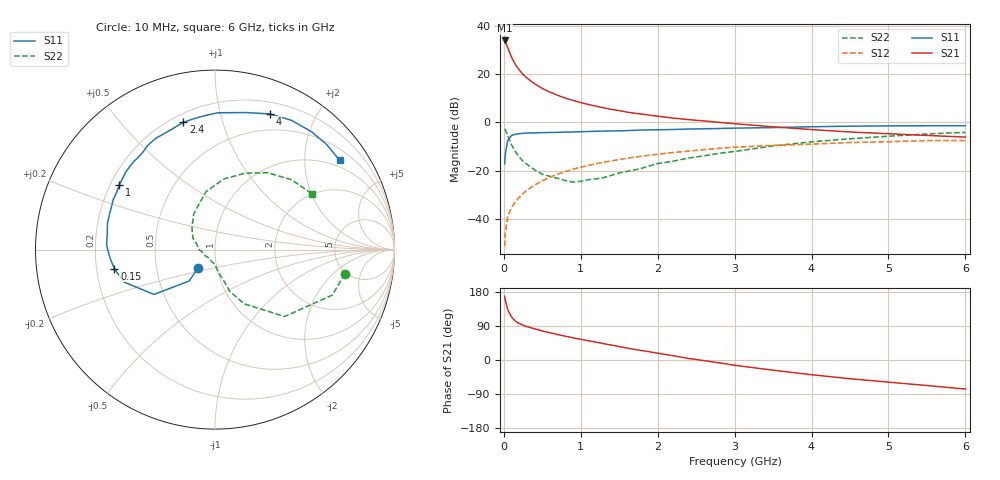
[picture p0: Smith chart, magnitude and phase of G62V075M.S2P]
! SIEMENS Small Signal Semiconductors
! BFG193
! Si NPN RF Bipolar Junction Transistor in SOT223
! VCE = 2 V  IC = 75 mA
! Common Emitter S-Parameters:  August  1996
# GHz  S  MA  R  50
!  f  S11  S21  S12  S22
! GHz  MAG  ANG  MAG  ANG  MAG  ANG  MAG  ANG
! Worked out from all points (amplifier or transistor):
!   36 points, 10 MHz to 6 GHz, reference 50 ohm
!   highest |S21| = 34.1 dB at 10 MHz (marker M1)
!   |S21| within 3 dB of that: start of sweep to 50.66 MHz
!   unconditionally stable (mu >= 1): start of sweep to 18.9 MHz; 178.8 MHz to 2.977 GHz; 3.075 GHz to 3.645 GHz
!   at 250 MHz: K = 1.06, MAG = 23.3 dB, |S12| = -29.5 dB
!   at 1.4 GHz: K = 1.11, MAG = 8.7 dB, |S12| = -16.0 dB
!   at 6 GHz: K = 1.00, MSG = 0.7 dB, |S12| = -7.5 dB
!   S11 on the Smith chart (normalised r, x): 10 MHz: 0.81, -0.17; 150 MHz: 0.28, -0.09; 1 GHz: 0.24, +0.29; 2.4 GHz: 0.25, +0.75; 4 GHz: 0.32, +1.43; 6 GHz: 0.79, +2.92
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0.01  0.1376 -132.7  50.46 168.0  0.0027 73.3  0.7358 -10.5
0.02  0.2262 -129.4  47.25 157.3  0.0052 72.5  0.701 -21.2
0.05  0.422 -143.7  35.94 132.8  0.0112 63.2  0.5379 -43.9
0.1  0.5383 -160.4  22.73 113.3  0.0171 64.5  0.3431 -61.7
0.15  0.5708 -169.3  15.97 102.5  0.0225 65.2  0.2467 -70.5
0.2  0.5852 -174.9  12.34 96.5  0.0278 66.9  0.1937 -73.1
0.25  0.5959 -179.2  9.963 91.8  0.0334 67.6  0.1557 -77.1
0.3  0.6044 177.4  8.381 88.2  0.0391 68.9  0.1357 -80.1
0.4  0.6069 171.3  6.34 82.3  0.0502 69.4  0.1035 -85.2
0.5  0.6166 166.4  5.086 76.6  0.0615 68.2  0.0843 -89.8
0.6  0.6197 161.9  4.269 71.8  0.0732 67.0  0.0758 -95.8
0.8  0.6317 154.0  3.21 62.7  0.0956 63.4  0.0622 -116.4
1  0.6438 145.8  2.589 54.5  0.1176 59.5  0.06 -136.4
1.1  0.6496 142.4  2.362 50.7  0.1282 57.7  0.0649 -147.5
1.6  0.6775 125.9  1.644 31.6  0.18 46.1  0.0966 171.9
2.2  0.7144 109.0  1.233 11.3  0.2373 31.7  0.1567 143.8
2.4  0.7307 103.9  1.146 4.3  0.2546 27.3  0.1828 134.5
3.5  0.7828 77.3  0.813 -26.9  0.3337 -0.9  0.3254 99.1
4  0.8154 68.0  0.713 -38.8  0.3554 -10.8  0.3969 82.9
4.5  0.8372 59.3  0.634 -49.4  0.3832 -21.1  0.4585 68.3
5.5  0.8544 43.3  0.538 -67.4  0.421 -44.4  0.5771 42.5
6  0.8543 35.6  0.497 -76.7  0.4213 -57.7  0.6232 29.9
